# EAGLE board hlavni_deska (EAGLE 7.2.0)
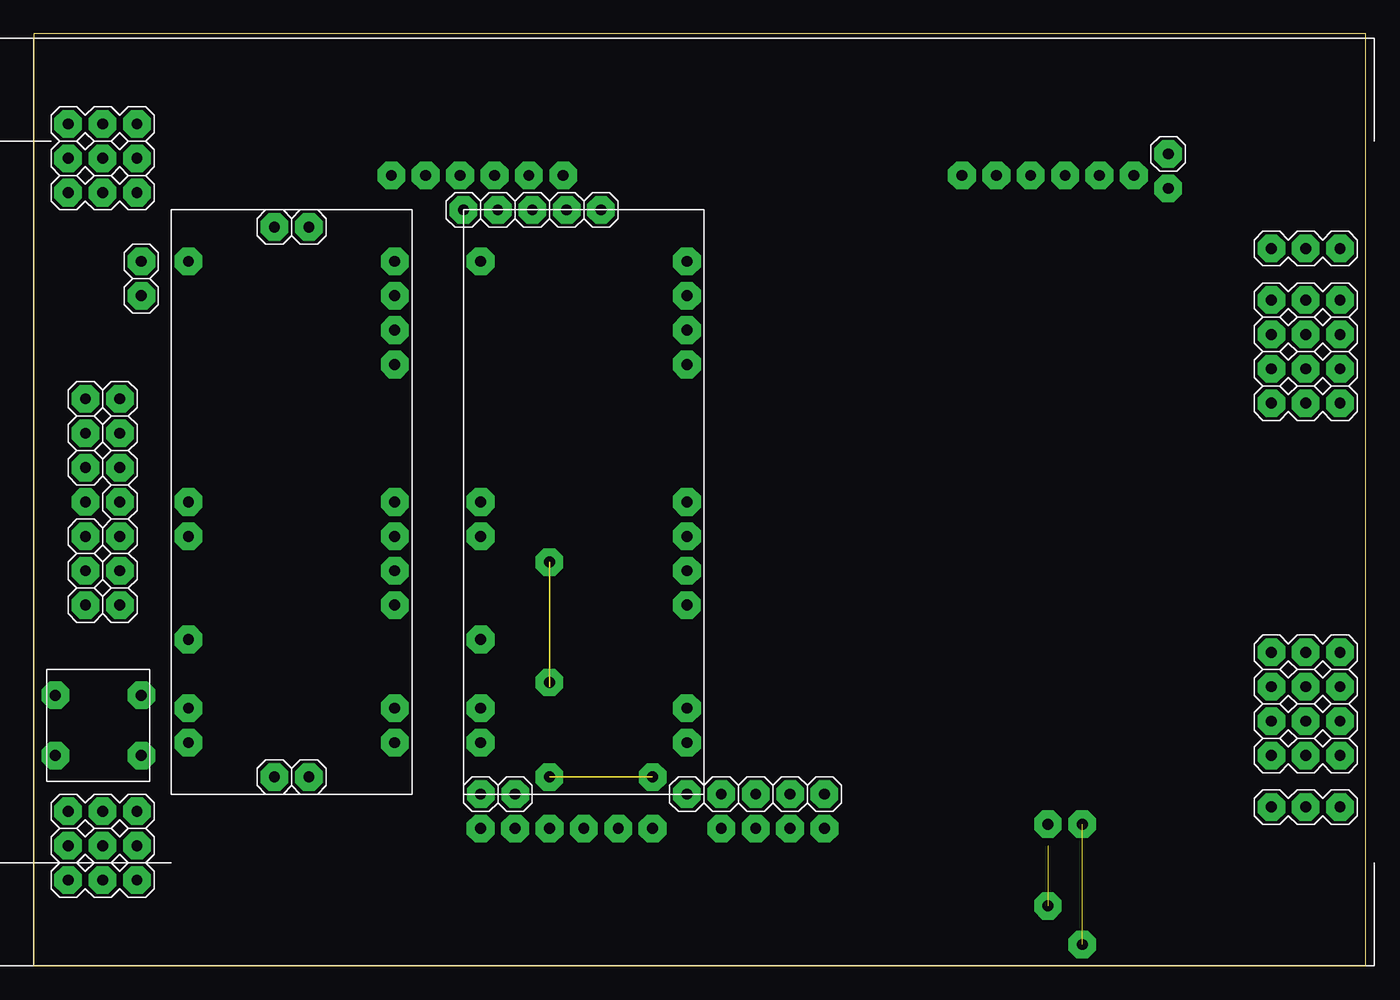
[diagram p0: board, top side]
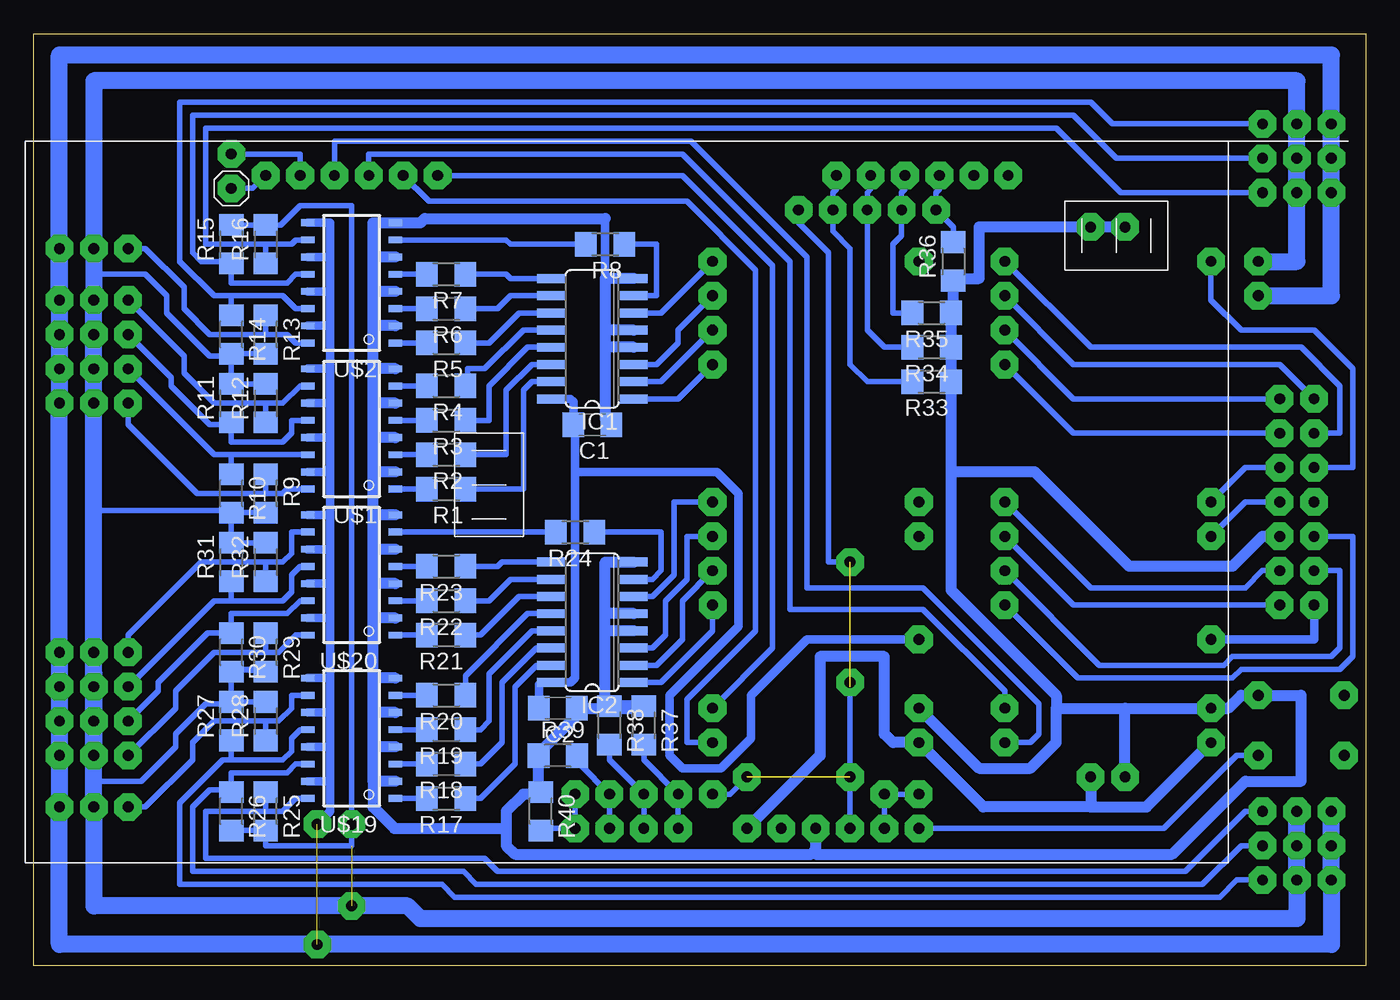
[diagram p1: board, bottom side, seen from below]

Size 98.41 x 68.89 mm. Coordinates in mm from the lower left corner, seen from the top.
Outline: 0,0 98.41,0 98.41,68.89 0,68.89 0,0
Copper layers (1*16): Top 0.035mm / dielectric 1.5mm / Bottom 0.035mm
Design rules "default": minimum track width 10mil, minimum drill 24mil, track to track 8mil, track to pad 8mil, pad to pad 8mil, via to via 8mil, smd to smd 8mil, copper to edge 40mil, drill to drill 8mil, minimum pad ring 10mil, minimum via ring 8mil, stop-mask expansion 4mil, vias tented up to drill 0mil, thermal gap 10mil

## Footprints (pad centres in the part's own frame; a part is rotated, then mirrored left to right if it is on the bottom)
C1206 = smd 1.6 x 1.8: 1 -1.4,0; 2 1.4,0
SO16 = smd 0.66 x 2.032: 1 -4.445,-3.073; 2 -3.175,-3.073; 3 -1.905,-3.073; 4 -0.635,-3.073; 5 0.635,-3.073; 6 1.905,-3.073; 7 3.175,-3.073; 8 4.445,-3.073; 9 4.445,3.073; 10 3.175,3.073; 11 1.905,3.073; 12 0.635,3.073; 13 -0.635,3.073; 14 -1.905,3.073; 15 -3.175,3.073; 16 -4.445,3.073
R1206 = smd 1.6 x 1.803: 1 -1.422,0; 2 1.422,0
MINI-FLAT-16 = smd 1 x 0.5: 1 -3.24,4.445; 2 -3.24,3.175; 3 -3.24,1.905; 4 -3.24,0.635; 5 -3.24,-0.635; 6 -3.24,-1.905; 7 -3.24,-3.175; 8 -3.24,-4.445; 9 3.24,-4.445; 10 3.24,-3.175; 11 3.24,-1.905; 12 3.24,-0.635; 13 3.24,0.635; 14 3.24,1.905; 15 3.24,3.175; 16 3.24,4.445
MOJE_1 = drill 0.8 pad 2.032 octagon: P$1 0,0
MEGA = drill 0.8 pad 2.05 octagon: P$1 33.02,10.16; P$4 35.56,10.16; P$5 38.1,10.16; P$6 40.64,10.16; P$7 43.18,10.16; P$8 45.72,10.16; P$19 50.8,10.16; P$20 53.34,10.16; P$21 55.88,10.16; P$22 58.42,10.16; P$63 81.28,58.42; P$64 78.74,58.42; P$65 76.2,58.42; P$66 73.66,58.42; P$67 71.12,58.42; P$68 68.58,58.42; P$80 26.416,58.42; P$81 28.956,58.42; P$82 31.496,58.42; P$83 34.036,58.42; P$84 36.576,58.42; P$85 39.116,58.42
NANO = drill 0.8 pad 2.05 octagon: P$1 1.27,3.81; P$3 1.27,6.35; P$5 1.27,11.43; P$8 1.27,19.05; P$9 1.27,21.59; P$16 1.27,39.37; P$17 16.51,3.81; P$18 16.51,6.35; P$24 16.51,16.51; P$25 16.51,19.05; P$26 16.51,21.59; P$28 16.51,31.75; P$29 16.51,34.29; P$30 16.51,36.83; P$31 16.51,39.37 | drill 0.8 pad 2.032 octagon: P$4 16.51,13.97
MOJE_3 = drill 0.8 pad 2.032 octagon: P$1 -2.54,0; P$2 0,0; P$3 2.54,0
CON_1 = drill 0.8 pad 2.032 octagon: P$1 0,0
BUT = drill 0.8 pad 2.032 octagon: P$1 1.905,0.635; P$2 6.35,0.635; P$3 1.905,6.985; P$4 6.35,6.985

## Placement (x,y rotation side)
C1  [C1206]  57.15,40.01 180 bottom
C2  [C1206]  59.69,19.05 180 bottom
IC1  74AC138D  [SO16]  57.15,46.35 90 bottom
IC2  74AC138D  [SO16]  57.15,25.4 90 bottom
R1  [R1206]  67.94,35.24 180 bottom
R2  [R1206]  67.94,37.78 180 bottom
R3  [R1206]  67.94,40.32 180 bottom
R4  [R1206]  67.94,42.86 180 bottom
R5  [R1206]  67.94,46.04 180 bottom
R6  [R1206]  67.94,48.58 180 bottom
R7  [R1206]  67.94,51.12 180 bottom
R8  [R1206]  56.2,53.34 180 bottom
R9  [R1206]  81.28,34.92 270 bottom
R10  [R1206]  83.82,34.92 270 bottom
R11  [R1206]  83.82,41.59 90 bottom
R12  [R1206]  81.28,41.59 90 bottom
R13  [R1206]  81.28,46.67 270 bottom
R14  [R1206]  83.82,46.67 270 bottom
R15  [R1206]  83.82,53.34 90 bottom
R16  [R1206]  81.28,53.34 90 bottom
R17  [R1206]  67.94,12.38 180 bottom
R18  [R1206]  67.94,14.92 180 bottom
R19  [R1206]  67.94,17.46 180 bottom
R20  [R1206]  67.94,20 180 bottom
R21  [R1206]  67.94,24.45 180 bottom
R22  [R1206]  67.94,26.99 180 bottom
R23  [R1206]  67.94,29.53 180 bottom
R24  [R1206]  58.42,32.07 180 bottom
R25  [R1206]  81.28,11.43 270 bottom
R26  [R1206]  83.82,11.43 270 bottom
R27  [R1206]  83.82,18.1 90 bottom
R28  [R1206]  81.28,18.1 90 bottom
R29  [R1206]  81.28,23.18 270 bottom
R30  [R1206]  83.82,23.18 270 bottom
R31  [R1206]  83.82,29.84 90 bottom
R32  [R1206]  81.28,29.84 90 bottom
R33  [R1206]  32.07,43.18 180 bottom
R34  [R1206]  32.07,45.72 180 bottom
R35  [R1206]  32.07,48.26 180 bottom
R36  [R1206]  30.48,52.07 90 bottom
R37  [R1206]  53.34,17.78 270 bottom
R38  [R1206]  55.88,17.78 270 bottom
R39  [R1206]  59.69,15.56 0 bottom
R40  [R1206]  60.96,11.43 270 bottom
U$1  TLP281-4  [MINI-FLAT-16]  74.93,39.69 180 bottom
U$2  TLP281-4  [MINI-FLAT-16]  74.93,50.48 180 bottom
U$3  GND2  [MOJE_1]  7.94,49.53 0 top
U$4  MEGA  [MEGA]  0,0 0 top
U$5  NANO  [NANO]  10.16,12.7 0 top
U$6  SRV1  [MOJE_3]  93.98,41.59 180 top
U$7  SRV2  [MOJE_3]  93.98,44.13 180 top
U$8  SRV3  [MOJE_3]  93.98,46.67 180 top
U$9  SRV4  [MOJE_3]  93.98,49.21 180 top
U$10  SRV5  [MOJE_3]  93.98,53.02 180 top
U$11  SRV6  [MOJE_3]  5.08,62.23 0 top
U$12  SRV7  [MOJE_3]  5.08,59.69 0 top
U$13  SRV8  [MOJE_3]  5.08,57.15 0 top
U$14  NANO  [NANO]  31.75,12.7 0 top
U$17  Vcc2  [MOJE_1]  7.94,52.07 0 top
U$19  TLP281-4  [MINI-FLAT-16]  74.93,16.83 180 bottom
U$20  TLP281-4  [MINI-FLAT-16]  74.93,28.89 180 bottom
U$24  SRV1  [MOJE_3]  5.08,11.43 0 top
U$25  SRV2  [MOJE_3]  5.08,8.89 0 top
U$26  SRV3  [MOJE_3]  5.08,6.35 0 top
U$27  SRV4  [MOJE_3]  93.98,11.75 180 top
U$28  SRV5  [MOJE_3]  93.98,15.56 180 top
U$29  SRV6  [MOJE_3]  93.98,18.1 180 top
U$30  SRV7  [MOJE_3]  93.98,20.64 180 top
U$31  SRV8  [MOJE_3]  93.98,23.18 180 top
U$38  ECHO  [CON_1]  3.81,29.21 0 top
U$39  TRIG  [CON_1]  6.35,29.21 0 top
U$42  ECHO  [CON_1]  6.35,26.67 0 top
U$43  TRIG  [CON_1]  3.81,36.83 0 top
U$46  ECHO  [CON_1]  3.81,39.37 0 top
U$47  TRIG  [CON_1]  3.81,41.91 0 top
U$50  ECHO  [CON_1]  6.35,41.91 0 top
U$51  TRIG  [CON_1]  6.35,39.37 0 top
U$52  5V  [CON_1]  3.81,26.67 90 top
U$53  GND  [CON_1]  20.32,54.61 0 top
U$54  SDA  [CON_1]  6.35,34.29 0 top
U$55  SCL  [CON_1]  6.35,36.83 0 top
U$56  INT  [CON_1]  3.81,31.75 0 top
U$57  3.3V  [CON_1]  35.56,12.7 0 top
U$58  3.3V  [CON_1]  33.02,12.7 0 top
U$59  GND  [CON_1]  6.35,31.75 0 top
U$60  GND  [CON_1]  17.78,54.61 0 top
U$61  RX  [CON_1]  83.82,60.01 0 top
U$62  TX  [CON_1]  83.82,57.47 0 bottom
U$63  GND  [CON_1]  17.78,13.97 0 top
U$65  BUTTON  [BUT]  8.57,13.65 90 top
U$66  Vin  [CON_1]  20.32,13.97 0 top
U$68  BUTTON  [CON_1]  39.37,55.88 0 top
U$69  5V  [CON_1]  48.26,12.7 0 top
U$70  BUTTON  [CON_1]  36.83,55.88 0 top
U$71  BUTTON  [CON_1]  34.29,55.88 270 top
U$72  BUTTON  [CON_1]  31.75,55.88 0 top
U$73  BUTTON  [CON_1]  50.8,12.7 0 top
U$74  5V  [CON_1]  41.91,55.88 0 top
U$75  BUTTON  [CON_1]  53.34,12.7 0 top
U$76  BUTTON  [CON_1]  55.88,12.7 0 top
U$77  BUTTON  [CON_1]  58.42,12.7 0 top

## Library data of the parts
C1 C2 R1-R40 = rcl
IC1 IC2 = 74xx-eu
U$1 U$2 U$19 U$20 = optocoupler
U$3 U$6-U$13 U$17 U$24-U$31 = con-lstb
U$4 U$5 U$14 U$38 U$39 U$42 U$43 U$46 U$47 U$50-U$63 U$65 U$66 U$68-U$77 = arduino

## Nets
N$1: R9.1 U$1.16 U$6.P$3
N$2: R10.1 U$1.14 U$7.P$3
N$3: R11.1 U$1.12 U$8.P$3
N$4: R12.1 U$1.10 U$9.P$3
N$5: R13.1 U$2.16 U$10.P$3
N$6: R14.1 U$2.14 U$11.P$3
N$7: R15.1 U$2.12 U$12.P$3
N$8: R16.1 U$2.10 U$13.P$3
N$9 [GND2]: U$1.9 U$1.11 U$1.13 U$1.15 U$2.9 U$2.11 U$2.13 U$2.15 U$3.P$1 U$6.P$1 U$7.P$1 U$8.P$1 U$9.P$1 U$10.P$1 U$11.P$1 U$12.P$1 U$13.P$1 U$19.9 U$19.11 U$19.13 U$19.15 U$20.9 U$20.11 U$20.13 U$20.15 U$24.P$1 U$25.P$1 U$26.P$1 U$27.P$1 U$28.P$1 U$29.P$1 U$30.P$1 U$31.P$1
N$10: U$5.P$31 U$46.P$1
N$11: U$5.P$30 U$47.P$1
N$12: R1.2 U$1.1
N$13: R2.2 U$1.3
N$14: R3.2 U$1.5
N$15: R4.2 U$1.7
N$16: R5.2 U$2.1
N$17: R6.2 U$2.3
N$18: R7.2 U$2.5
N$19: R8.2 U$2.7
N$20: R40.2 U$4.P$22 U$77.P$1
N$21: U$5.P$29 U$50.P$1
N$22: IC1.12 R4.1
N$23: IC1.13 R3.1
N$24: IC1.14 R2.1
N$25: IC1.15 R1.1
N$26: IC1.11 R5.1
N$27: IC1.10 R6.1
N$28: U$4.P$8 U$5.P$1 U$14.P$1 U$66.P$1
N$29: IC1.7 R8.1
N$30: IC1.1 U$14.P$28
N$31: IC1.2 U$14.P$29
N$32: IC1.3 U$14.P$30
N$33: R25.1 U$19.16 U$24.P$3
N$34: IC1.6 U$14.P$31
N$35: R26.1 U$19.14 U$25.P$3
N$36: R27.1 U$19.12 U$26.P$3
N$37: R28.1 U$19.10 U$27.P$3
N$38: R29.1 U$20.16 U$28.P$3
N$39: R30.1 U$20.14 U$29.P$3
N$40: R31.1 U$20.12 U$30.P$3
N$41: R32.1 U$20.10 U$31.P$3
N$42: U$5.P$28 U$51.P$1
N$43 [VCC2]: R9.2 R10.2 R11.2 R12.2 R13.2 R14.2 R15.2 R16.2 R25.2 R26.2 R27.2 R28.2 R29.2 R30.2 R31.2 R32.2 U$6.P$2 U$7.P$2 U$8.P$2 U$9.P$2 U$10.P$2 U$11.P$2 U$12.P$2 U$13.P$2 U$17.P$1 U$24.P$2 U$25.P$2 U$26.P$2 U$27.P$2 U$28.P$2 U$29.P$2 U$30.P$2 U$31.P$2
N$44: R17.2 U$19.1
N$45: R18.2 U$19.3
N$46: R19.2 U$19.5
N$47: R20.2 U$19.7
N$48: R21.2 U$20.1
N$49: R22.2 U$20.3
N$50: R23.2 U$20.5
N$51: R24.2 U$20.7
N$52: U$5.P$16 U$43.P$1
N$53: IC2.12 R20.1
N$54: IC2.13 R19.1
N$55: IC2.14 R18.1
N$56: IC2.15 R17.1
N$57: IC2.11 R21.1
N$59: IC1.9 R7.1
N$60: IC2.7 R24.1
N$61: IC2.6 U$14.P$26
N$62: IC2.3 U$14.P$25
N$63: IC2.2 U$14.P$24
N$64: IC2.1 U$14.P$4
N$65: C1.2 C2.2 IC1.16 IC2.16 U$14.P$5
N$66: U$5.P$25 U$42.P$1
N$67: U$5.P$26 U$39.P$1
N$68: U$5.P$24 U$38.P$1
N$69: U$5.P$8 U$54.P$1
N$70: U$5.P$9 U$55.P$1
N$71: U$5.P$4 U$56.P$1
N$72: U$5.P$5 U$52.P$1
N$73: C1.1 C2.1 IC1.4 IC1.5 IC1.8 IC2.4 IC2.5 IC2.8 R33.1 R34.1 R35.1 R36.1 R37.1 R38.1 R39.1 R40.1 U$1.2 U$1.4 U$1.6 U$1.8 U$2.2 U$2.4 U$2.6 U$2.8 U$4.P$6 U$5.P$3 U$14.P$3 U$19.2 U$19.4 U$19.6 U$19.8 U$20.2 U$20.4 U$20.6 U$20.8 U$53.P$1 U$59.P$1 U$60.P$1 U$63.P$1 U$65.P$2
N$74: IC2.9 R23.1
N$77: IC2.10 R22.1
N$78: U$4.P$65 U$5.P$17
N$79: U$4.P$66 U$5.P$18
N$80: U$4.P$68 U$14.P$18
N$81: U$4.P$67 U$14.P$17
N$82: R39.2 U$4.P$21 U$76.P$1
N$83: R38.2 U$4.P$20 U$75.P$1
N$84: R37.2 U$4.P$19 U$73.P$1
N$85: R36.2 U$4.P$82 U$72.P$1
N$86: R35.2 U$4.P$83 U$71.P$1
N$87: R34.2 U$4.P$84 U$70.P$1
N$88: R33.2 U$4.P$85 U$68.P$1
N$89: U$4.P$1 U$65.P$1
N$90: U$4.P$4 U$57.P$1 U$58.P$1
N$91: U$4.P$5 U$69.P$1 U$74.P$1
N$92: U$4.P$63 U$62.P$1
N$93: U$4.P$64 U$61.P$1

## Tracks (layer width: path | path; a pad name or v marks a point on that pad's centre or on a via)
N$1
  Bottom 0.406: U$1.16 79.69,35.24 80.01,34.92 81.28,34.92 | 81.28,34.92 86.36,34.92 91.44,40.01 U$6.P$3 | R9.1 81.28,34.92
N$2
  Bottom 0.406: 83.82,37.78 R10.1 | U$1.14 83.82,37.78 | 83.82,37.78 85.09,37.78 U$7.P$3
N$3
  Bottom 0.406: U$1.12 79.38,40.32 79.38,39.37 80.01,38.73 83.82,38.73 R11.1 83.99,40.01 85.41,40.01 88.27,42.86 88.27,43.5 U$8.P$3
N$4
  Bottom 0.406: 81.28,41.59 85.09,41.59 87.31,43.81 87.31,45.09 U$9.P$3 | 81.28,41.59 80.01,41.59 78.74,42.86 U$1.10 | R12.1 81.28,41.59
N$5
  Bottom 0.406: U$2.16 79.06,46.04 79.69,46.67 81.28,46.67 | 81.28,46.67 R13.1 | U$10.P$3 90.17,53.02 87.31,50.16 87.31,48.58 85.41,46.67 81.28,46.67
N$6
  Bottom 0.406: R14.1 83.82,49.53 | 83.82,49.53 80.01,49.53 79.06,48.58 U$2.14 | 83.82,49.53 85.09,49.53 87.63,52.07 87.63,63.82 20.32,63.82 18.73,62.23 U$11.P$3
N$7
  Bottom 0.406: U$2.12 79.06,51.12 79.69,50.48 83.82,50.48 R15.1 83.97,52.07 86.04,52.07 86.68,52.7 86.68,62.87 21.59,62.87 18.41,59.69 U$12.P$3
N$8
  Bottom 0.406: 81.28,53.34 R16.1 | U$2.10 79.06,53.66 79.38,53.34 81.28,53.34 | 81.28,53.34 85.72,53.34 85.72,61.91 22.86,61.91 18.1,57.15 U$13.P$3
N$9  (via drill 0.8 pad 2.03)  (1 unrouted)
  Bottom 0.406: U$9.P$1 U$27.P$1
  Bottom 0.61: U$2.9 76.52,54.93 76.52,52.39 | 76.52,52.39 76.52,49.85 | 76.52,49.85 76.52,47.31 | 76.52,47.31 76.52,44.13 | 76.52,44.13 76.52,41.59 | 76.52,41.59 76.52,39.05 | 76.52,39.05 76.52,36.83 | 76.52,36.83 76.52,33.34 | 76.52,33.34 76.52,30.8 | 76.52,30.8 76.52,28.26 | 76.52,28.26 76.52,25.72 | 76.52,25.72 76.52,21.27 | 76.52,21.27 76.52,18.73 | 76.52,18.73 76.52,16.19 | 76.52,16.19 76.52,13.65 | 76.52,13.65 76.52,11.43 77.47,10.48 | U$19.15 76.52,13.65 | U$19.13 76.52,16.19 | U$19.11 76.52,18.73 | U$19.9 76.52,21.27 | U$20.15 76.52,25.72 | U$20.13 76.52,28.26 | U$20.11 76.52,30.8 | U$20.9 76.52,33.34 | U$1.15 76.83,36.51 76.52,36.83 | U$1.13 76.52,39.05 | U$1.11 76.52,41.59 | U$1.9 76.52,44.13 | U$2.15 76.52,47.31 | U$2.13 76.52,49.85 | U$2.11 76.52,52.39
  Bottom 1.27: U$10.P$1 U$9.P$1 | U$9.P$1 U$8.P$1 U$7.P$1 U$6.P$1 U$31.P$1 U$30.P$1 U$29.P$1 U$28.P$1 U$27.P$1 96.52,1.59 v77.47,1.59 2.54,1.59 U$26.P$1 U$25.P$1 U$24.P$1 | U$9.P$1 96.52,67.31 2.54,67.31 U$13.P$1 | U$13.P$1 U$12.P$1 U$11.P$1 | U$3.P$1 2.54,49.53 U$13.P$1
N$10
  Bottom 0.406: U$5.P$31 20.32,45.72 4.76,45.72 1.91,42.86 1.91,39.37 U$46.P$1
N$11
  Bottom 0.406: U$47.P$1 6.35,44.45 21.59,44.45 U$5.P$30
N$12
  Bottom 0.406: R1.2 U$1.1
N$13
  Bottom 0.406: R2.2 U$1.3
N$14
  Bottom 0.406: R3.2 U$1.5
N$15
  Bottom 0.406: R4.2 U$1.7
N$16
  Bottom 0.406: R5.2 U$2.1
N$17
  Bottom 0.406: R6.2 U$2.3
N$18
  Bottom 0.406: R7.2 U$2.5
N$19
  Bottom 0.406: R8.2 63.18,53.34 63.5,53.66 U$2.7
N$20
  Bottom 0.406: U$77.P$1 U$4.P$22 60.96,10.16 R40.2
N$21
  Bottom 0.406: U$5.P$29 21.59,41.91 U$50.P$1
N$22
  Bottom 0.406: IC1.12 62.23,46.99 65.09,44.13 66.36,44.13 66.36,43.03 R4.1
N$23
  Bottom 0.406: R3.1 64.77,40.32 64.77,42.86 61.91,45.72 IC1.13
N$24
  Bottom 0.406: R2.1 63.5,37.78 63.5,42.55 61.59,44.45 IC1.14
N$25
  Bottom 0.406: R1.1 62.23,35.24 62.23,42.55 61.59,43.18 IC1.15
N$26
  Bottom 0.406: R5.1 64.77,46.04 62.55,48.26 IC1.11
N$27
  Bottom 0.406: IC1.10 63.18,49.53 64.14,48.58 R6.1
N$28
  Bottom 0.813: 20.32,11.75 28.26,11.75 U$14.P$1 34.92,16.51 35.56,17.14 35.56,22.86 40.32,22.86 40.32,15.56 U$4.P$8 | U$66.P$1 20.32,11.75 | 20.32,11.75 16.19,11.75 U$5.P$1
N$29
  Bottom 0.406: IC1.7 52.39,49.53 52.39,53.34 R8.1
N$30
  Bottom 0.406: IC1.1 50.8,41.91 U$14.P$28
N$31
  Bottom 0.406: IC1.2 52.07,43.18 U$14.P$29
N$32
  Bottom 0.406: U$14.P$30 50.8,46.99 50.8,46.04 52.39,44.45 IC1.3
N$33
  Bottom 0.406: U$24.P$3 8.89,11.43 13.34,6.99 64.14,6.99 65.09,7.94 85.72,7.94 85.72,11.43 81.28,11.43 | 81.28,11.43 R25.1 | U$19.16 79.06,12.38 80.01,11.43 81.28,11.43
N$34
  Bottom 0.406: U$14.P$31 52.07,48.26 IC1.6
N$35
  Bottom 0.406: U$19.14 79.06,14.92 79.69,14.29 83.82,14.29 83.82,13.02 | 83.82,13.02 85.41,13.02 86.68,11.75 86.68,6.99 66.67,6.99 65.72,6.03 12.06,6.03 9.21,8.89 U$25.P$3 | R26.1 83.82,13.02
N$36
  Bottom 0.406: U$19.12 78.74,17.46 79.38,16.83 79.38,15.88 80.01,15.24 83.82,15.24 | 83.82,15.24 R27.1 | 83.82,15.24 84.45,15.24 87.63,12.06 87.63,6.03 68.26,6.03 67.31,5.08 10.79,5.08 9.53,6.35 U$26.P$3
N$37
  Bottom 0.406: R28.1 81.28,18.1 | 81.28,18.1 80.33,18.1 79.38,19.05 79.38,20 U$19.10 | 81.28,18.1 85.09,18.1 86.68,16.51 86.68,15.24 90.17,11.75 U$27.P$3
N$38
  Bottom 0.406: 81.28,23.18 80.33,23.18 79.06,24.45 U$20.16 | U$28.P$3 87.95,19.05 87.95,20.32 85.09,23.18 81.28,23.18 | R29.1 81.28,23.18
N$39
  Bottom 0.406: U$20.14 78.74,26.99 79.69,26.04 83.82,26.04 R30.1 85.57,24.6 89.22,20.95 89.22,20.32 U$29.P$3
N$40
  Bottom 0.406: 83.82,26.99 80.01,26.99 79.38,27.62 79.38,28.89 78.74,29.53 U$20.12 | 83.82,26.99 R31.1 83.97,28.42 | U$30.P$3 85.09,26.99 83.82,26.99
N$41
  Bottom 0.406: U$20.10 79.38,32.07 79.38,30.48 80.01,29.84 81.28,29.84 | 81.28,29.84 86.04,29.84 91.44,24.45 U$31.P$3 | R32.1 81.28,29.84
N$42
  Bottom 0.406: U$51.P$1 21.59,39.37 U$5.P$28
N$43  (via drill 0.8 pad 2.03)  (1 unrouted)
  Bottom 0.406: R28.2 R27.2 | R29.2 83.82,21.91 | 83.82,31.43 R31.2 R32.2 83.34,31.27 83.5,31.43 83.82,31.43 | R10.2 83.82,33.66 93.98,33.66 | R10.2 R9.2 | R13.2 R14.2 83.82,45.09 | R12.2 R11.2 83.82,45.09 | 83.82,31.43 R10.2 | R15.2 R16.2 80.17,54.76 78.74,56.2 74.93,56.2 v74.93,10.48 74.93,8.89 81.28,8.89 R25.2 R26.2 | 83.82,45.09 85.41,45.09 88.58,48.26 88.58,49.53 90.17,51.12 93.98,51.12 | 81.43,21.91 83.82,21.91 | 93.98,13.65 90.49,13.65 87.95,16.19 87.95,17.14 85.72,19.37 83.82,19.37 R27.2 | R27.2 R30.2 83.82,21.91
  Bottom 1.27: U$9.P$2 U$8.P$2 U$7.P$2 U$6.P$2 93.98,33.66 U$28.P$2 | U$9.P$2 93.98,51.12 U$10.P$2 93.98,65.41 5.08,65.41 U$13.P$2 | 93.98,46.04 U$9.P$2 | U$28.P$2 93.98,13.65 U$27.P$2 93.98,4.45 v74.93,4.45 70.8,4.45 69.85,3.49 5.08,3.49 U$26.P$2 U$25.P$2 U$24.P$2 | 93.98,21.59 U$28.P$2 | U$28.P$2 U$29.P$2 U$30.P$2 U$31.P$2 | U$13.P$2 U$12.P$2 U$11.P$2 | U$17.P$1 5.08,52.07 U$13.P$2
N$44
  Bottom 0.406: R17.2 U$19.1
N$45
  Bottom 0.406: R18.2 U$19.3
N$46
  Bottom 0.406: R19.2 U$19.5
N$47
  Bottom 0.406: R20.2 U$19.7
N$48
  Bottom 0.406: R21.2 U$20.1
N$49
  Bottom 0.406: R22.2 U$20.3
N$50
  Bottom 0.406: R23.2 U$20.5
N$51
  Bottom 0.406: R24.2 U$20.7
N$52
  Bottom 0.406: U$43.P$1 0.95,36.83 0.95,44.13 3.81,46.99 9.21,46.99 11.43,49.21 U$5.P$16
N$53
  Bottom 0.406: IC2.12 61.91,26.04 66.52,21.42 R20.1
N$54
  Bottom 0.406: IC2.13 61.59,24.77 64.77,21.59 64.77,18.1 65.41,17.46 R19.1
N$55
  Bottom 0.406: IC2.14 61.28,23.5 63.82,20.95 63.82,16.51 65.41,14.92 R18.1
N$56
  Bottom 0.406: IC2.15 61.28,22.23 62.87,20.64 62.87,14.92 65.41,12.38 R17.1
N$57
  Bottom 0.406: IC2.11 62.55,27.3 65.41,24.45 R21.1
N$58  (via drill 0.8 pad 2.03)
  other vias: 77.47,10.48
N$59
  Bottom 0.406: R7.1 63.5,51.12 63.18,50.8 IC1.9
N$60
  Bottom 0.406: R24.1 52.07,32.07 52.07,29.21 52.7,28.57 IC2.7
N$61
  Bottom 0.406: IC2.6 52.7,27.3 51.12,28.89 51.12,34.29 U$14.P$26
N$62
  Bottom 0.406: IC2.3 52.7,23.5 51.75,24.45 51.75,26.99 50.16,28.57 50.16,31.75 U$14.P$25
N$63
  Bottom 0.406: IC2.2 52.39,22.23 50.48,24.13 50.48,26.99 U$14.P$24
N$64
  Bottom 0.406: IC2.1 52.07,20.95 48.26,24.77 U$14.P$4
N$65
  Bottom 0.406: C1.2 58.42,40.01
  Bottom 0.61: U$14.P$5 41.27,24.13 45.4,20 45.4,16.83 47.62,14.61 50.48,14.61 51.44,15.56 51.44,20 46.35,25.08 46.35,34.92 47.94,36.51 58.42,36.51 | 58.42,36.51 58.42,39.88 C1.2 58.55,41.72 58.74,41.91 IC1.16 | 58.42,36.51 58.42,21.27 58.74,20.95 IC2.16 60.96,20.95 61.09,20.82 C2.2
N$66
  Bottom 0.406: U$5.P$25 21.59,26.67 U$42.P$1
N$67
  Bottom 0.406: U$5.P$26 20.32,27.94 8.89,27.94 7.62,29.21 U$39.P$1
N$68
  Bottom 0.406: U$38.P$1 1.91,29.21 1.91,23.5 2.54,22.86 9.84,22.86 10.48,22.23 19.68,22.23 U$5.P$24
N$69
  Bottom 0.406: U$5.P$8 8.89,34.29 U$54.P$1
N$70
  Bottom 0.406: U$5.P$9 8.89,36.83 U$55.P$1
N$71
  Bottom 0.406: U$56.P$1 0.95,31.75 0.95,22.86 1.91,21.91 9.21,21.91 9.84,21.27 21.27,21.27 U$5.P$4
N$72
  Bottom 0.61: U$5.P$5 3.81,24.13 U$52.P$1
N$73
  Bottom 0.406: 56.03,19.05 56.52,19.05 56.36,19.2 R38.1 | 30.48,48.42 R35.1 30.48,48.26 | R34.1 30.48,45.72 | R33.1 30.48,43.18 | 61.11,12.7 R40.1 | R39.1 60.96,15.56 | C2.1 58.42,19.05
  Bottom 0.61: 56.2,55.24 56.2,50.8
  Bottom 0.813: U$14.P$3 28.57,14.61 24.77,14.61 22.86,16.51 22.86,19.05 | 22.86,19.05 17.78,19.05 | 17.78,19.05 U$5.P$3 10.16,19.05 9.21,20 U$65.P$2 4.76,20 4.76,13.65 8.89,13.65 14.29,8.26 40.64,8.26 40.64,8.57 | U$60.P$1 U$53.P$1 28.57,54.61 28.57,50.8 30.33,50.8 R36.1 30.48,48.42 | R35.1 R34.1 | R34.1 R33.1 | U$4.P$6 40.64,8.57 | 60.96,15.56 60.96,15.88 58.42,18.41 58.42,18.92 C2.1 56.52,19.05 53.49,19.05 R37.1 56.03,19.2 56.2,19.37 56.2,24.77 | IC2.4 56.2,24.77 | 56.2,24.77 56.2,26.04 | IC2.5 56.2,26.04 | 56.2,26.04 56.2,29.84 IC2.8 | 61.11,12.85 60.96,12.7 62.23,12.7 63.5,11.43 63.5,10.16 | 63.5,10.16 63.5,8.89 62.87,8.26 40.96,8.26 40.64,8.57 | 61.11,12.85 R39.1 | 61.11,12.85 R40.1 | 73.34,13.65 73.34,16.19 | 73.34,16.19 73.34,18.73 | 73.34,18.73 73.34,21.27 | 73.34,21.27 73.34,25.72 | 73.34,25.72 73.34,28.26 | 73.34,28.26 73.34,30.8 | 73.34,30.8 73.34,33.34 | 73.34,33.34 73.34,36.51 | 73.34,36.51 73.34,39.37 | 73.34,39.37 73.34,41.59 | 73.34,41.59 73.34,44.13 | 73.34,44.13 73.34,47.31 | 73.34,47.31 73.34,49.85 | 73.34,49.85 73.34,52.39 | 73.34,52.39 73.34,54.93 U$2.8 69.85,54.93 69.53,55.24 56.2,55.24 | IC1.8 56.2,50.8 56.2,46.99 | IC1.5 56.2,46.99 | 56.2,46.99 56.2,45.72 | IC1.4 56.2,45.72 | 56.2,45.72 56.2,40.45 C1.1 | U$19.2 73.34,13.65 | 73.34,13.65 73.34,11.75 71.75,10.16 63.5,10.16 | U$19.4 73.34,16.19 | U$19.6 73.34,18.73 | U$19.8 73.34,21.27 | U$20.2 73.34,25.72 | U$20.4 73.34,28.26 | U$20.6 73.34,30.8 | U$20.8 73.34,33.34 | U$1.2 73.34,36.51 | U$1.4 73.03,39.05 73.34,39.37 | U$1.6 73.34,41.59 | U$1.8 73.34,44.13 | U$2.2 73.34,47.31 | U$2.4 73.34,49.85 | U$2.6 73.34,52.39 | R34.1 30.64,36.2 | 30.64,36.2 30.64,27.79 22.86,20 22.86,19.05
  Bottom 0.813: U$63.P$1 17.78,19.05 | U$59.P$1 7.62,31.75 9.84,29.53 17.46,29.53 24.45,36.51 30.33,36.51 30.64,36.2
N$74
  Bottom 0.406: IC2.9 63.82,29.84 64.14,29.53 R23.1
N$75  (via drill 0.8 pad 2.03)
  other vias: 3.81,34.29
N$76  (via drill 0.8 pad 2.03)
  other vias: 45.72,13.97
N$77
  Bottom 0.406: R22.1 64.77,26.99 63.18,28.57 IC2.10
N$78
  Bottom 0.406: U$5.P$17 24.77,16.51 24.13,17.14 24.13,19.37 32.7,27.94 41.27,27.94 41.27,52.39 49.85,60.96 76.2,60.96 U$4.P$65
N$79
  Bottom 0.406: U$4.P$66 73.66,60.01 50.48,60.01 42.55,52.07 42.55,26.35 32.7,26.35 26.67,20.32 U$5.P$18
N$80
  Bottom 0.406: U$14.P$18 43.81,23.5 43.81,51.75 50.48,58.42 U$4.P$68
N$81
  Bottom 0.406: U$4.P$67 69.22,56.52 50.16,56.52 45.09,51.44 45.09,24.77 50.16,19.68 50.16,16.51 U$14.P$17
N$82
  Bottom 0.406: U$4.P$21 U$76.P$1 58.1,14.92 58.1,15.39 R39.2
N$83
  Bottom 0.406: U$4.P$20 U$75.P$1 55.88,15.24 R38.2
N$84
  Bottom 0.406: U$4.P$19 U$73.P$1 53.34,15.24 R37.2
N$85
  Bottom 0.406: R36.2 30.48,54.61 U$72.P$1 31.75,57.15 31.5,57.4 U$4.P$82
N$86
  Bottom 0.406: U$4.P$83 34.04,57.4 34.29,57.15 U$71.P$1 34.29,53.98 34.92,53.34 34.92,48.26 R35.2
N$87
  Bottom 0.406: U$4.P$84 36.58,57.4 36.83,57.15 U$70.P$1 36.83,46.99 35.56,45.72 R34.2
N$88
  Bottom 0.406: U$4.P$85 39.12,57.4 39.37,57.15 U$68.P$1 39.37,54.29 38.1,53.02 38.1,44.45 36.83,43.18 R33.2
N$89
  Bottom 0.406: U$65.P$1 9.53,15.56 14.92,10.16 U$4.P$1
N$90
  Bottom 0.406: U$4.P$4 U$57.P$1 U$58.P$1
N$91  (via drill 0.8 pad 2.03)  (8 unrouted)
  Bottom 0.406: U$74.P$1 41.91,54.93 39.69,52.7 39.69,29.84 v38.1,29.84 | v38.1,20.95 v38.1,13.97 U$4.P$5 | U$69.P$1 46.99,12.7 45.72,13.97
N$92
  Bottom 0.406: U$4.P$63 82.23,57.47 U$62.P$1
N$93
  Bottom 0.406: 78.74,58.74 U$4.P$64 78.74,60.01 U$61.P$1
